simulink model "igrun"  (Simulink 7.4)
settings: Solver=ode45  StartTime=0  StopTime=30  MaxStep=1e-3  RelTol=1e-3
undefined symbols (not defined in the file or in its folder): wmo
libraries: simulink_extras x1, mrlib x1

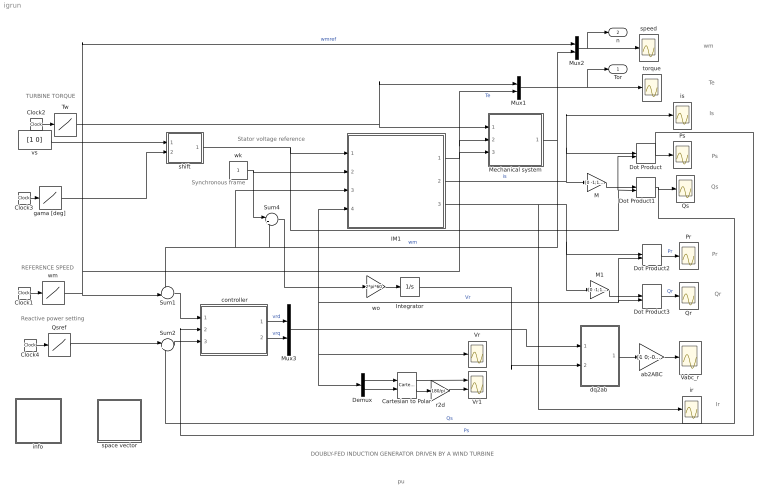
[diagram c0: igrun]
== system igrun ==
  note: Reactive power setting
  note: TURBINE TORQUE
  note: REFERENCE SPEED
  note: Synchronous frame
  note: Stator voltage reference
  note: DOUBLY-FED INDUCTION GENERATOR DRIVEN BY A WIND TURBINE
  note: pu
  note: Ps
  note: Qs
  note: Pr
  note: Qr
  note: Ir
  note: Is
  note: Te
  note: wm
  " controller" : Subsystem  mask{Kpn=8, Kin=10, Kpt=2, Kit=1, KpQ=.5, KiQ=8, sat=2}
      mask prompts: Kpn "Proportional gain of speed loop"; Kin "Integral gain of speed loop"; Kpt "Proportional gain of torque loop"; Kit "Integral gain of torque loop"; KpQ "Proportional gain of Qs loop"; KiQ "Integral gain of Qs loop"; sat "Saturation limit [pu]"
      mask help: PI controllers for speed, Ps, and Qs
  Cartesian to Polar : simulink_extras/Transformations/Cartesian to Polar  SystemSampleTime=-1
  Clock{1..4} (4 alike) : Clock
  Demux : Demux  Outputs=2
  Dot Product{,1..3} (4 alike) : DotProduct  OutDataType=fixdt(1, 16)  OutScaling=2^-10
  IM1 : Subsystem  mask{Rs=0.05, Lsl=0.1, Rr=0.02, Lm=5, Lrl=0.1, wo=2*pi*60}
      mask prompts: Rs "Stator resistance [pu]"; Lsl "Stator leakage inductance [pu]"; Rr "Rotor resistance [pu]"; Lm "Magnetizing inductance [pu]"; Lrl "Rotor leakage inductance [pu]"; wo "base frequency [rad/s]"
      mask help: Induction Machine
  Integrator : Integrator
  M : Gain  Gain=[0 -1;1 0]  Multiplication=Matrix(K*u)  ParameterDataType=sfix(16)  ParameterScaling=2^0  OutDataType=sfix(16)  OutScaling=2^0
  M1 : Gain  Gain=[0 -1;1 0]  Multiplication=Matrix(K*u)  ParameterDataType=sfix(16)  ParameterScaling=2^0  OutDataType=sfix(16)  OutScaling=2^0
  Mechanical system : Subsystem  mask{Hw=2.5, Hg=0.5, Km=.4}
      mask prompts: Hw "Turbine inertia constant [s]"; Hg "Generator inertia constant [s]"; Km "Shaft compliance constant [pu/rad]"
      mask help: Mechanical System
  Mux1 : Mux  Inputs=2
  Mux2 : Mux  Inputs=2
  Mux3 : Mux  Inputs=2
  Pr : Scope
  Ps : Scope
  Qr : Scope
  Qs : Scope
  Qsref : Lookup  InputValues=[0 5 5.01 30 ]  Table=[0 0 -.5 -.5 ]  OutDataType=sfix(16)  OutScaling=2^0
  Sum1 : Sum  Inputs=-+|  OutDataType=sfix(16)  OutScaling=2^0
  Sum2 : Sum  Inputs=|+-  OutDataType=sfix(16)  OutScaling=2^0
  Sum4 : Sum  Inputs=|+-  OutDataType=sfix(16)  OutScaling=2^0
  Tw : Lookup  InputValues=[0 5 5.01 30 ]  Table=[0 0 -1 -1]  OutDataType=sfix(16)  OutScaling=2^0
  Vabc_r : Scope
  Vr : Scope
  Vr1 : Scope  NumInputPorts=2
  ab2ABC : Gain  Gain=[1 0;-0.5 sqrt(3)/2;-0.5 -sqrt(3)/2]  Multiplication=Matrix(K*u)  ParameterDataType=sfix(16)  ParameterScaling=2^0  OutDataType=sfix(16)  OutScaling=2^0
  "dq2ab " : Subsystem
  gama [deg] : Lookup  InputValues="[0  50]"  Table=[0 0]  OutDataType=sfix(16)  OutScaling=2^0
  info : Subsystem
  ir : Scope
  is : Scope
  r2d : Gain  Gain=180/pi  Multiplication=Matrix(K*u)  ParameterDataType=sfix(16)  ParameterScaling=2^0  OutDataType=sfix(16)  OutScaling=2^0
  shift : Subsystem
  space vector : Subsystem
  speed : Scope
  torque : Scope
  vs : Constant  Value=[1 0]  OutDataType=sfix(16)  OutScaling=2^0
  wk : Constant  OutDataType=sfix(16)  OutScaling=2^0
  wm : Lookup  InputValues=[0 15 16 30 ]  Table=[.7 .7 1.3 1.3 ]  OutDataType=sfix(16)  OutScaling=2^0
  wo : Gain  Gain=2*pi*60  ParameterDataType=sfix(16)  ParameterScaling=2^0  OutDataType=sfix(16)  OutScaling=2^0
  Tor : Outport
  n : Outport  Port=2
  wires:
  wk/1 -> IM1/2(wk), Sum4/1
  Dot Product/1 -> Ps/1, " controller"/2(Ps)  "Ps"
  M/1 -> Dot Product1/1
  IM1/1(Te) -> Mechanical system/2(Te), Mux1/2  "Te"
  Clock2/1 -> Tw/1
  Tw/1 -> Mux1/1, Mechanical system/1(Tw)
  Dot Product1/1 -> Qs/1, Sum2/2  "Qs"
  Mux1/1 -> torque/1, Tor/1
  IM1/2(is) -> M/1, Dot Product/1, is/1  "is"
  Dot Product2/1 -> Pr/1  "Pr"
  M1/1 -> Dot Product3/1
  Dot Product3/1 -> Qr/1  "Qr"
  IM1/3(ir) -> M1/1, Dot Product2/1, ir/1
  Mechanical system/1(wm) -> Mux2/2, Sum1/1, IM1/3(wm), Sum4/2  "wm"
  wm/1 -> Sum1/2, Mechanical system/3(wmo), Mux2/1  "wmref"
  Mux2/1 -> speed/1, n/1
  Clock1/1 -> wm/1
  Sum2/1 -> " controller"/3(Qser)
  Clock3/1 -> gama [deg]/1
  shift/1(vs) -> Dot Product/2, Dot Product1/2, IM1/1(vs)
  vs/1 -> shift/1(vso)
  gama [deg]/1 -> shift/2(gama)
  Demux/1 -> Cartesian to Polar/1
  Demux/2 -> Cartesian to Polar/2
  Cartesian to Polar/1 -> Vr1/1
  Cartesian to Polar/2 -> r2d/1
  r2d/1 -> Vr1/2
  Mux3/1 -> IM1/4(vr), Dot Product3/2, Dot Product2/2, Demux/1, Vr/1, "dq2ab "/1(dq)  "Vr"
  "dq2ab "/1(ab) -> ab2ABC/1
  ab2ABC/1 -> Vabc_r/1
  wo/1 -> Integrator/1
  Sum4/1 -> wo/1
  Integrator/1 -> "dq2ab "/2(thetar)
  Clock4/1 -> Qsref/1
  Qsref/1 -> Sum2/1
  " controller"/1(vrd) -> Mux3/1  "vrd"
  " controller"/2(vrq) -> Mux3/2  "vrq"
  Sum1/1 -> " controller"/1(wmer)

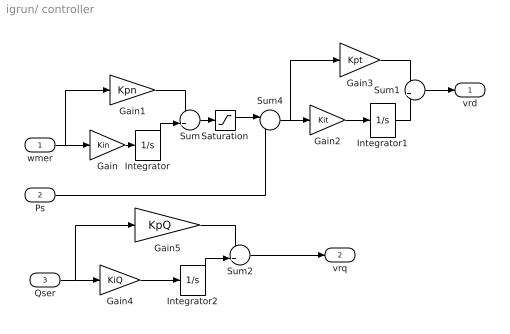
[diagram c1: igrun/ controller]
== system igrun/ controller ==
  wmer : Inport  OutDataType=sfix(16)  OutScaling=2^0
  Ps : Inport  Port=2  OutDataType=sfix(16)  OutScaling=2^0
  Qser : Inport  Port=3  OutDataType=sfix(16)  OutScaling=2^0
  Gain : Gain  Gain=Kin  ParameterDataType=sfix(16)  ParameterScaling=2^0  OutDataType=sfix(16)  OutScaling=2^0
  Gain1 : Gain  Gain=Kpn  ParameterDataType=sfix(16)  ParameterScaling=2^0  OutDataType=sfix(16)  OutScaling=2^0
  Gain2 : Gain  Gain=Kit  ParameterDataType=sfix(16)  ParameterScaling=2^0  OutDataType=sfix(16)  OutScaling=2^0
  Gain3 : Gain  Gain=Kpt  ParameterDataType=sfix(16)  ParameterScaling=2^0  OutDataType=sfix(16)  OutScaling=2^0
  Gain4 : Gain  Gain=KiQ  ParameterDataType=sfix(16)  ParameterScaling=2^0  OutDataType=sfix(16)  OutScaling=2^0
  Gain5 : Gain  Gain=KpQ  ParameterDataType=sfix(16)  ParameterScaling=2^0  OutDataType=sfix(16)  OutScaling=2^0
  Integrator : Integrator  LimitOutput=on  UpperSaturationLimit=sat  LowerSaturationLimit=-sat
  Integrator1 : Integrator  InitialCondition=0.306  UpperSaturationLimit=sat  LowerSaturationLimit=-sat
  Integrator2 : Integrator  InitialCondition=-0.0045  UpperSaturationLimit=sat  LowerSaturationLimit=-sat
  Saturation : Saturate  UpperLimit=sat  LowerLimit=-sat
  Sum : Sum  OutDataType=sfix(16)  OutScaling=2^0
  Sum1 : Sum  OutDataType=sfix(16)  OutScaling=2^0
  Sum2 : Sum  OutDataType=sfix(16)  OutScaling=2^0
  Sum4 : Sum  Inputs=|-+  OutDataType=sfix(16)  OutScaling=2^0
  vrd : Outport  InitialOutput=0
  vrq : Outport  Port=2  InitialOutput=0
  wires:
  Sum/1 -> Saturation/1
  wmer/1 -> Gain1/1, Gain/1
  Gain/1 -> Integrator/1
  Gain1/1 -> Sum/1
  Integrator/1 -> Sum/2
  Sum1/1 -> vrd/1
  Sum4/1 -> Gain2/1, Gain3/1
  Gain2/1 -> Integrator1/1
  Gain3/1 -> Sum1/1
  Integrator1/1 -> Sum1/2
  Saturation/1 -> Sum4/1
  Sum2/1 -> vrq/1
  Qser/1 -> Gain5/1, Gain4/1
  Gain4/1 -> Integrator2/1
  Gain5/1 -> Sum2/1
  Integrator2/1 -> Sum2/2
  Ps/1 -> Sum4/2

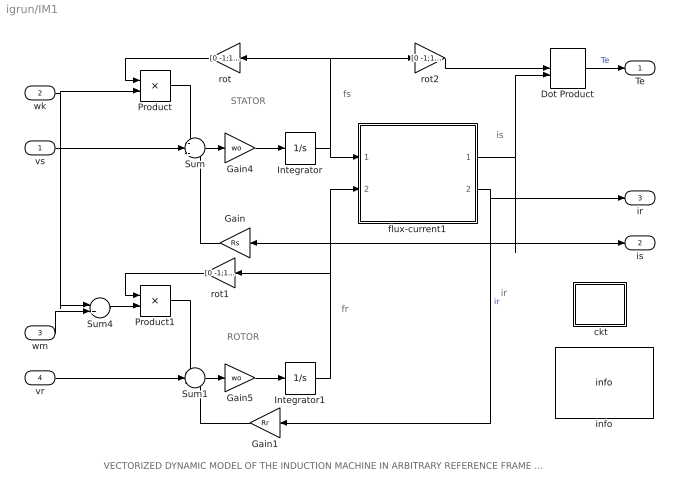
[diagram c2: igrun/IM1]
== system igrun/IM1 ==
  note: ROTOR
  note: STATOR
  note: fs
  note: fr
  note: is
  note: VECTORIZED DYNAMIC MODEL OF THE INDUCTION MACHINE IN ARBITRARY REFERENCE FRAME (per unit formulation)
  note: ir
  vs : Inport  OutDataType=sfix(16)  OutScaling=2^0
  wk : Inport  Port=2  OutDataType=sfix(16)  OutScaling=2^0
  wm : Inport  Port=3  OutDataType=sfix(16)  OutScaling=2^0
  vr : Inport  Port=4  OutDataType=sfix(16)  OutScaling=2^0
  " ckt" : Subsystem
  Dot Product : DotProduct  OutDataType=fixdt(1, 16)  OutScaling=2^-10
  Gain : Gain  Gain=Rs  ParameterDataType=sfix(16)  ParameterScaling=2^0  OutDataType=sfix(16)  OutScaling=2^0
  Gain1 : Gain  Gain=Rr  ParameterDataType=sfix(16)  ParameterScaling=2^0  OutDataType=sfix(16)  OutScaling=2^0
  Gain4 : Gain  Gain=wo  ParameterDataType=sfix(16)  ParameterScaling=2^0  OutDataType=sfix(16)  OutScaling=2^0
  Gain5 : Gain  Gain=wo  ParameterDataType=sfix(16)  ParameterScaling=2^0  OutDataType=sfix(16)  OutScaling=2^0
  Integrator : Integrator  InitialCondition=[0 -1]
  Integrator1 : Integrator  InitialCondition=[0 -1.02]
  Product : Product  OutDataType=sfix(16)  OutScaling=2^0
  Product1 : Product  OutDataType=sfix(16)  OutScaling=2^0
  Sum : Sum  Inputs=-+-  OutDataType=sfix(16)  OutScaling=2^0
  Sum1 : Sum  Inputs=-+-  OutDataType=sfix(16)  OutScaling=2^0
  Sum4 : Sum  Inputs=|+-  OutDataType=sfix(16)  OutScaling=2^0
  flux-current1 : Subsystem
  info : mrlib/IM/info  SystemSampleTime=-1
  rot : Gain  Gain=[0 -1;1 0]  Multiplication=Matrix(K*u)  ParameterDataType=sfix(16)  ParameterScaling=2^0  OutDataType=sfix(16)  OutScaling=2^0
  rot1 : Gain  Gain=[0 -1;1 0]  Multiplication=Matrix(K*u)  ParameterDataType=sfix(16)  ParameterScaling=2^0  OutDataType=sfix(16)  OutScaling=2^0
  rot2 : Gain  Gain=[0 -1;1 0]  Multiplication=Matrix(K*u)  ParameterDataType=sfix(16)  ParameterScaling=2^0  OutDataType=sfix(16)  OutScaling=2^0
  Te : Outport
  is : Outport  Port=2
  ir : Outport  Port=3
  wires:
  Gain/1 -> Sum/3
  Gain1/1 -> Sum1/3
  flux-current1/2(ir) -> Gain1/1, ir/1  "ir"
  Integrator/1 -> flux-current1/1(fs), rot/1, rot2/1
  Integrator1/1 -> flux-current1/2(fr), rot1/1
  Product1/1 -> Sum1/1
  rot1/1 -> Product1/1
  Product/1 -> Sum/1
  rot/1 -> Product/1
  rot2/1 -> Dot Product/1
  Sum4/1 -> Product1/2
  Sum/1 -> Gain4/1
  Gain4/1 -> Integrator/1
  Sum1/1 -> Gain5/1
  Gain5/1 -> Integrator1/1
  flux-current1/1(is) -> Gain/1, is/1, Dot Product/2
  Dot Product/1 -> Te/1  "Te"
  vs/1 -> Sum/2
  wk/1 -> Product/2, Sum4/1
  wm/1 -> Sum4/2
  vr/1 -> Sum1/2

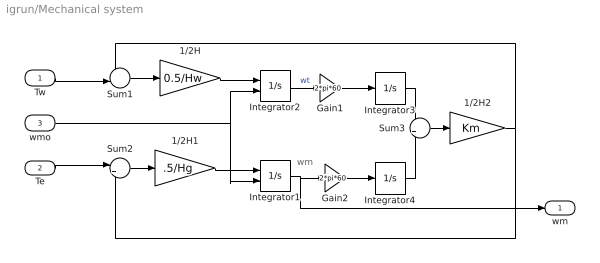
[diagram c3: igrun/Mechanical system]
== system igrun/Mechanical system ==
  note: wm
  Tw : Inport  OutDataType=sfix(16)  OutScaling=2^0
  Te : Inport  Port=2  OutDataType=sfix(16)  OutScaling=2^0
  wmo : Inport  Port=3  OutDataType=sfix(16)  OutScaling=2^0
  1/2H : Gain  Gain=0.5/Hw  ParameterDataType=sfix(16)  ParameterScaling=2^0  OutDataType=sfix(16)  OutScaling=2^0
  1/2H1 : Gain  Gain=.5/Hg  ParameterDataType=sfix(16)  ParameterScaling=2^0  OutDataType=sfix(16)  OutScaling=2^0
  1/2H2 : Gain  Gain=Km  ParameterDataType=sfix(16)  ParameterScaling=2^0  OutDataType=sfix(16)  OutScaling=2^0
  Gain1 : Gain  Gain=2*pi*60  ParameterDataType=sfix(16)  ParameterScaling=2^0  OutDataType=sfix(16)  OutScaling=2^0
  Gain2 : Gain  Gain=2*pi*60  ParameterDataType=sfix(16)  ParameterScaling=2^0  OutDataType=sfix(16)  OutScaling=2^0
  Integrator1 : Integrator  InitialConditionSource=external  InitialCondition=wmo
  Integrator2 : Integrator  InitialConditionSource=external  InitialCondition=wmo
  Integrator3 : Integrator
  Integrator4 : Integrator
  Sum1 : Sum  Inputs=+-|  OutDataType=sfix(16)  OutScaling=2^0
  Sum2 : Sum  Inputs=|+-  OutDataType=sfix(16)  OutScaling=2^0
  Sum3 : Sum  Inputs=-+  OutDataType=sfix(16)  OutScaling=2^0
  wm : Outport
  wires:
  Tw/1 -> Sum1/2
  Sum1/1 -> 1/2H/1
  Te/1 -> Sum2/1
  1/2H/1 -> Integrator2/1
  Sum2/1 -> 1/2H1/1
  1/2H1/1 -> Integrator1/1
  Integrator3/1 -> Sum3/1
  Sum3/1 -> 1/2H2/1
  1/2H2/1 -> Sum1/1, Sum2/2
  Gain1/1 -> Integrator3/1
  Integrator2/1 -> Gain1/1  "wt"
  Gain2/1 -> Integrator4/1
  Integrator4/1 -> Sum3/2
  Integrator1/1 -> Gain2/1, wm/1
  wmo/1 -> Integrator2/2, Integrator1/2

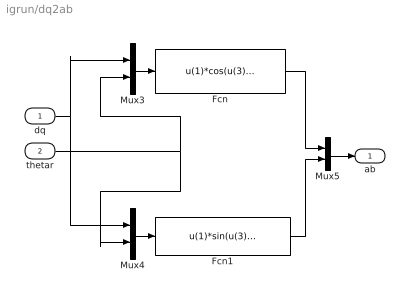
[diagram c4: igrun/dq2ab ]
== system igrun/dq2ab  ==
  dq : Inport  OutDataType=sfix(16)  OutScaling=2^0
  thetar : Inport  Port=2  OutDataType=sfix(16)  OutScaling=2^0
  Fcn : Fcn  Expr=u(1)*cos(u(3))-u(2)*sin(u(3))
  Fcn1 : Fcn  Expr=u(1)*sin(u(3))+u(2)*cos(u(3))
  Mux3 : Mux  Inputs=2
  Mux4 : Mux  Inputs=2
  Mux5 : Mux  Inputs=2
  ab : Outport
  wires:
  Mux3/1 -> Fcn/1
  Mux4/1 -> Fcn1/1
  dq/1 -> Mux3/1, Mux4/1
  thetar/1 -> Mux3/2, Mux4/2
  Fcn1/1 -> Mux5/2
  Fcn/1 -> Mux5/1
  Mux5/1 -> ab/1

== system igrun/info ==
  note: The induction machine is modeled in vectorized form in the synchronous frame associated with the stator voltage space vector. The dq components of the injected rotor voltage Vr, at slip frequency wr, are derived from PI controllers; vrd is the output of a cascade arrangement of speed and Ps controllers; vrq is derived from a Qs controller. The mechanical system is modeled as two inertias coupled by means of a flexible shaft. The whole system is described by parameters expressed in per unit. The machine representations are based on the motor convention; consequently, in the generator mode of operation, such quantities as Ps, Qs, Tw, Te are negative (with wm>0) while Pr is positive for subsynchronous operation and negative for oversynchronous mode.
  note: Doubly-Fed Induction Generator driven by a Wind Turbine

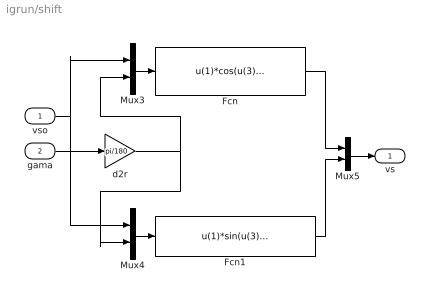
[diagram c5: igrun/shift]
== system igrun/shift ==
  vso : Inport  OutDataType=sfix(16)  OutScaling=2^0
  gama : Inport  Port=2  OutDataType=sfix(16)  OutScaling=2^0
  Fcn : Fcn  Expr=u(1)*cos(u(3))-u(2)*sin(u(3))
  Fcn1 : Fcn  Expr=u(1)*sin(u(3))+u(2)*cos(u(3))
  Mux3 : Mux  Inputs=2
  Mux4 : Mux  Inputs=2
  Mux5 : Mux  Inputs=2
  d2r : Gain  Gain=pi/180  Multiplication=Matrix(K*u)  ParameterDataType=sfix(16)  ParameterScaling=2^0  OutDataType=sfix(16)  OutScaling=2^0
  vs : Outport
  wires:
  Mux5/1 -> vs/1
  Fcn/1 -> Mux5/1
  Fcn1/1 -> Mux5/2
  gama/1 -> d2r/1
  vso/1 -> Mux4/1, Mux3/1
  Mux4/1 -> Fcn1/1
  Mux3/1 -> Fcn/1
  d2r/1 -> Mux4/2, Mux3/2

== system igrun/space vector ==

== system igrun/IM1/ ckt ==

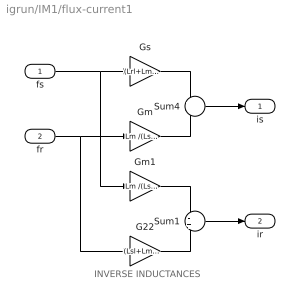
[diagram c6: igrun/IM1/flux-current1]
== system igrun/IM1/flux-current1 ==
  note: INVERSE INDUCTANCES
  fs : Inport  OutDataType=sfix(16)  OutScaling=2^0
  fr : Inport  Port=2  OutDataType=sfix(16)  OutScaling=2^0
  G22 : Gain  Gain=(Lsl+Lm )/(Lsl*Lrl+Lsl*Lm+Lrl*Lm)  ParameterDataType=sfix(16)  ParameterScaling=2^0  OutDataType=sfix(16)  OutScaling=2^0
  Gm : Gain  Gain=Lm /(Lsl*Lrl+Lsl*Lm+Lrl*Lm)  ParameterDataType=sfix(16)  ParameterScaling=2^0  OutDataType=sfix(16)  OutScaling=2^0
  Gm1 : Gain  Gain=Lm /(Lsl*Lrl+Lsl*Lm+Lrl*Lm)  ParameterDataType=sfix(16)  ParameterScaling=2^0  OutDataType=sfix(16)  OutScaling=2^0
  Gs : Gain  Gain=(Lrl+Lm) /(Lsl*Lrl+Lsl*Lm+Lrl*Lm)  ParameterDataType=sfix(16)  ParameterScaling=2^0  OutDataType=sfix(16)  OutScaling=2^0
  Sum1 : Sum  Inputs=-+  OutDataType=sfix(16)  OutScaling=2^0
  Sum4 : Sum  Inputs=+-  OutDataType=sfix(16)  OutScaling=2^0
  is : Outport
  ir : Outport  Port=2
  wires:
  fs/1 -> Gs/1, Gm1/1
  Gs/1 -> Sum4/1
  fr/1 -> Gm/1, G22/1
  Gm/1 -> Sum4/2
  Sum4/1 -> is/1
  Gm1/1 -> Sum1/1
  G22/1 -> Sum1/2
  Sum1/1 -> ir/1
